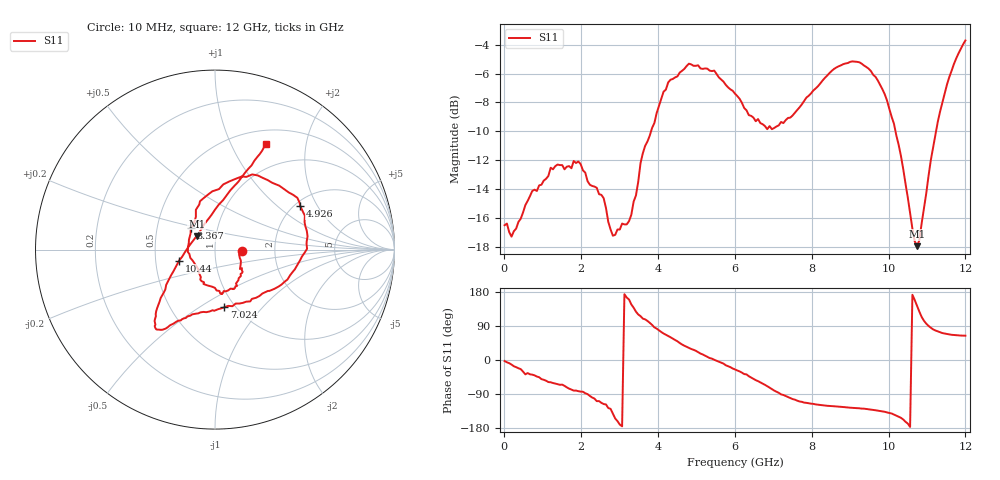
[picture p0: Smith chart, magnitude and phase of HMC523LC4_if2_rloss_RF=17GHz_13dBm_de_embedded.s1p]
!Hittite Microwave Corporation
!20 Alpha Rd
!Chelmsford, MA 01824
!Tel: 978-250-3343
!Fax: 978-250-3373
!Device: HMC523LC4, 0.01-12 GHz, GaAs MMIC Double-Balanced Mixer
!Misc: IF2 Return Loss with RF=17GHz at 13 dBm, Room
# MHZ S MA R 50
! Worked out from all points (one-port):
!   201 points, 10 MHz to 12 GHz, reference 50 ohm
!   lowest |S11| = -17.9 dB at 10.74 GHz (marker M1), VSWR 1.29, Z = 40.4 + j6.29 ohm
!   |S11| at or under -10 dB: start of sweep to 3.82 GHz; 10.18 GHz to 11.23 GHz (1.053 GHz wide, 9.83 % of centre)
!   S11 on the Smith chart (normalised r, x): 10 MHz: 1.35, -0.02; 3.367 GHz: 0.74, +0.19; 4.926 GHz: 2.14, +1.45; 7.024 GHz: 0.89, -0.64; 10.44 GHz: 0.66, -0.08; 12 GHz: 0.67, +1.37
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10  0.15 -2.7
189.85  0.137 -12.1
729.4  0.197 -38.7
1508.75  0.242 -65.0
1928.4  0.249 -82.3
2348.05  0.204 -101.9
2587.85  0.186 -116.2
2827.65  0.138 -141.6
3007.5  0.145 -170.4
3247.3  0.155 159.7
3367.2  0.181 138.1
3726.9  0.292 103.1
4146.55  0.434 69.9
4506.25  0.49 49.4
4925.9  0.533 26.9
5465.45  0.513 0.5
6005  0.427 -24.8
7024.15  0.325 -80.6
7503.75  0.359 -103.1
9002.5  0.55 -125.9
9482.1  0.521 -130.2
9901.75  0.425 -136.7
10141.55  0.336 -144.1
10441.3  0.209 -163.0
10501.25  0.187 -167.8
10741.05  0.127 142.9
11340.55  0.37 73.1
12000  0.652 64.1
